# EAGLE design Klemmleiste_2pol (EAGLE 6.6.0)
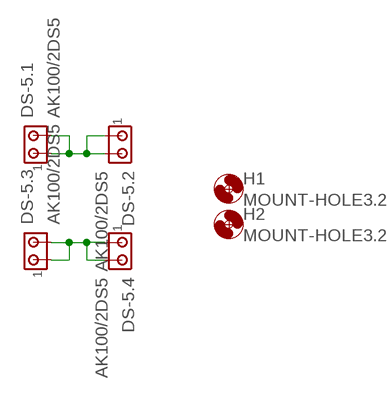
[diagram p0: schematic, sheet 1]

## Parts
DS-5.1  AK100/2DS5  [AK100/2DS-5.0-V]
DS-5.2  AK100/2DS5  [AK100/2DS-5.0-V]
DS-5.3  AK100/2DS5  [AK100/2DS-5.0-V]
DS-5.4  AK100/2DS5  [AK100/2DS-5.0-V]
H1  MOUNT-HOLE3.2  [3,2]
H2  MOUNT-HOLE3.2  [3,2]

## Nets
VDD: DS-5.1.1 DS-5.1.2 DS-5.2.1 DS-5.2.2
VSS: DS-5.3.1 DS-5.3.2 DS-5.4.1 DS-5.4.2

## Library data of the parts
DS-5.1-DS-5.4 = con_PTR:AK100/2: AK100/2
H1 H2 = holes:MOUNT-HOLE: MOUNTING HOLE with drill center marker

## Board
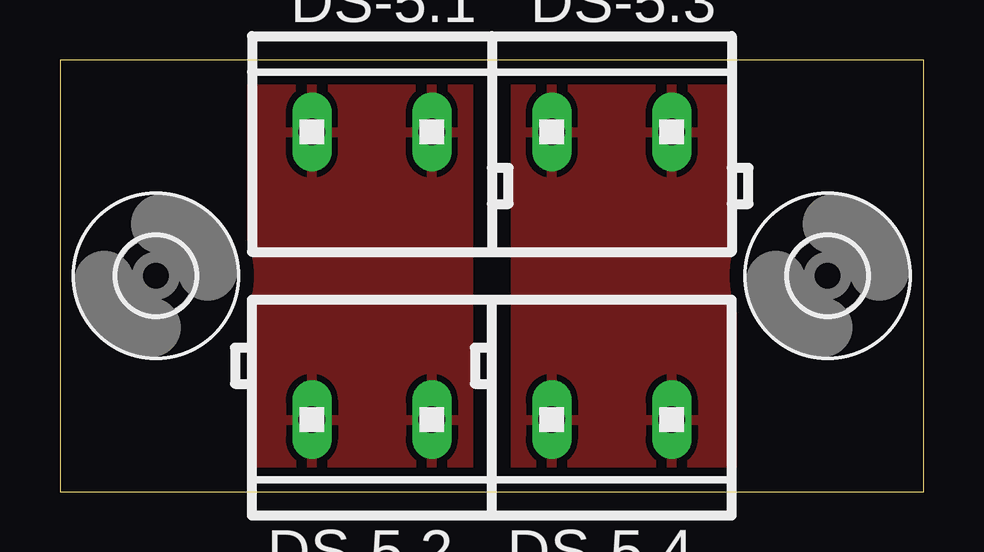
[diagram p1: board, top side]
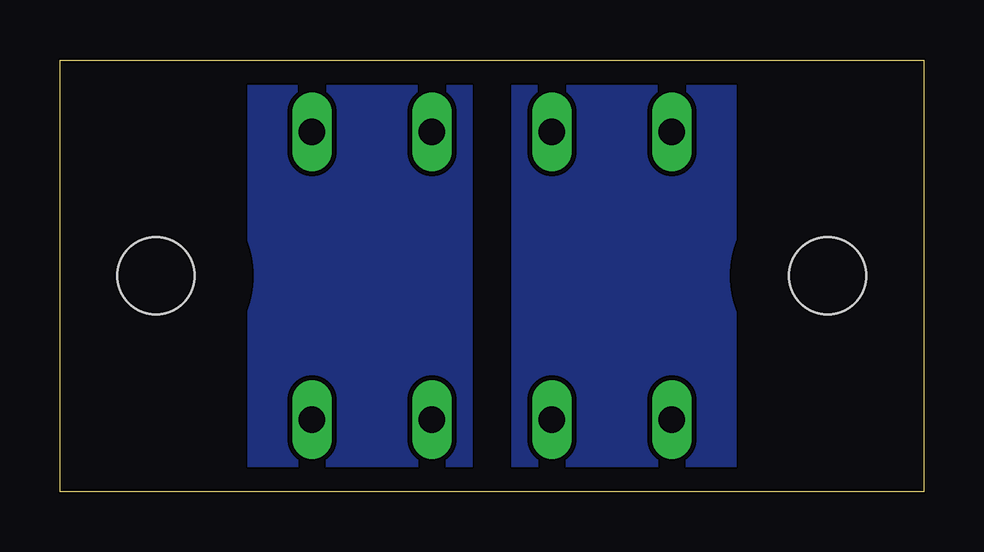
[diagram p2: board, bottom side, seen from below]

Size 36 x 18 mm. Coordinates in mm from the lower left corner, seen from the top.
Outline: 0,0 36,0 36,18 0,18 0,0
Copper layers (1*16): Top 0.035mm / dielectric 1.5mm / Bottom 0.035mm
Design rules "default": minimum track width 10mil, minimum drill 0.6mm, track to track 8mil, track to pad 8mil, pad to pad 8mil, via to via 8mil, smd to smd 8mil, copper to edge 40mil, drill to drill 8mil, minimum pad ring 10mil, minimum via ring 8mil, stop-mask expansion 4mil, vias tented up to drill 0mil, thermal gap 10mil

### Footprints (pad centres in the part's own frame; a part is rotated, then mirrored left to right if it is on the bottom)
AK100/2DS-5.0-V = drill 1.1 long: 1 -2.5,0; 2 2.5,0
3,2 = hole 3.2: 0,0

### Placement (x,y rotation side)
DS-5.1  13,15 180 top
DS-5.2  13,3 0 top
DS-5.3  23,15 180 top
DS-5.4  23,3 0 top
H1  4,9 0 top
H2  32,9 0 top

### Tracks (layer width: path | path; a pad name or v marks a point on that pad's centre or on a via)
VDD
  pour Top: 8,17 17,17 17,1 8,1
VDD1
  pour Bottom: 8,17 17,17 17,1 8,1
VSS
  pour Top: 19,17 28,17 28,1 19,1
VSS1
  pour Bottom: 19,17 28,17 28,1 19,1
